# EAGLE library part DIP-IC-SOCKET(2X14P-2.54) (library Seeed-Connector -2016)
320070000
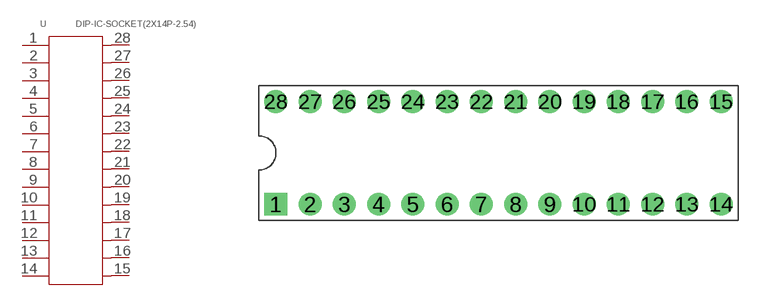
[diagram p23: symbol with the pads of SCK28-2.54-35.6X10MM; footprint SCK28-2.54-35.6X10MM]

Designator prefix U

## DIP-IC-SOCKET(2X14P-2.54) (MPN: ICX-28P; VALUE: 2x14p-2.54)  [SCK28-2.54-35.6X10MM]
1  1
2  2
3  3
4  4
5  5
6  6
7  7
8  8
9  9
10  10
11  11
12  12
13  13
14  14
15  15
16  16
17  17
18  18
19  19
20  20
21  21
22  22
23  23
24  24
25  25
26  26
27  27
28  28

## Footprint SCK28-2.54-35.6X10MM (pad centres in mm)
drill 1 pad 1.7 square: 1 -16.51,-3.81
drill 1 pad 1.7: 2 -13.97,-3.81; 3 -11.43,-3.81; 4 -8.89,-3.81; 5 -6.35,-3.81; 6 -3.81,-3.81; 7 -1.27,-3.81; 8 1.27,-3.81; 9 3.81,-3.81; 10 6.35,-3.81; 11 8.89,-3.81; 12 11.43,-3.81; 13 13.97,-3.81; 14 16.51,-3.81; 15 16.51,3.81; 16 13.97,3.81; 17 11.43,3.81; 18 8.89,3.81; 19 6.35,3.81; 20 3.81,3.81; 21 1.27,3.81; 22 -1.27,3.81; 23 -3.81,3.81; 24 -6.35,3.81; 25 -8.89,3.81; 26 -11.43,3.81; 27 -13.97,3.81; 28 -16.51,3.81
